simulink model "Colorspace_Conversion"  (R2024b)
settings: Solver=VariableStepAuto  StartTime=0.0  StopTime=10  RelTol=1e-3  EnableMultiTasking=on
undefined symbols (not defined in the file or in its folder): gray
libraries: ModelComposer x21, dspvision x1

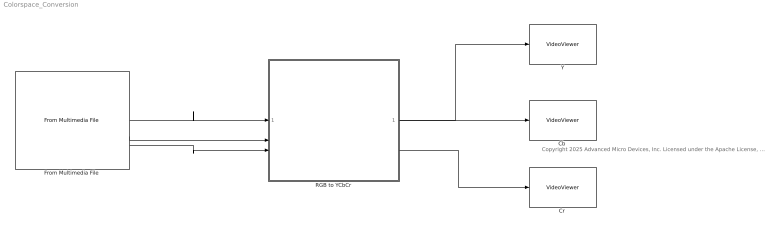
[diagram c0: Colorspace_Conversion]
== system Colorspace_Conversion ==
  note: Copyright 2025 Advanced Micro Devices, Inc. Licensed under the Apache License, Version 2.0 (the "License"); you may not use this file except in compliance with the License. You may obtain a copy of the License at http://www.apache.org/licenses/LICENSE-2.0 Unless required by applicable law or agreed to in writing, software distributed under the License is distributed on an "AS IS" BASIS, WITHOUT WARRANTIES OR CONDITIONS OF ANY KIND, either express or implied. See the License for the specific language governing permissions and limitations under the License.
  "Cb " : VideoViewer  colormapValue=gray(256)  FigPos=[23.4 519.6 487.2 356]
  "Cr " : VideoViewer  colormapValue=gray(256)  FigPos=[534.6 513.2 460.8 352]
  From Multimedia File : dspvision/From Multimedia File  inputFilename=visionface.avi  readRange=[1 Inf]  loop=on  numPlays=inf  outputStreams=Video only  videoDataType=single  audioDataType=int16  inheritSampleTime=on  userDefinedSampleTime=1/30  noAudioOutput=off  isIntensityVideo=off  fourcc=RGB  colorVideoFormat=Separate color signals  outputEOF=off  dataOrg=Column-major  audioFrameSize=1024  computeAudioFrameSize=off  outSamplingMode=Sample based
  RGB to YCbCr : Subsystem
  Y : VideoViewer  colormapValue=gray(256)  FigPos=[1016.2 530.8 471.2 368.8]
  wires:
  From Multimedia File/2 -> RGB to YCbCr/2(G)
  From Multimedia File/3 -> RGB to YCbCr/3(B)
  From Multimedia File/1 -> RGB to YCbCr/1(R)
  RGB to YCbCr/1(Y) -> Y/1
  RGB to YCbCr/2(Cb) -> "Cb "/1
  RGB to YCbCr/3(Cr) -> "Cr "/1

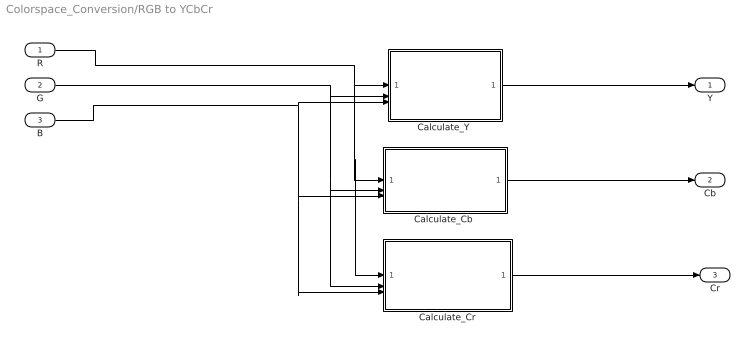
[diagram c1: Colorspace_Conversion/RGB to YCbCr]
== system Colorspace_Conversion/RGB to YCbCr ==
  R : Inport
  G : Inport  Port=2
  B : Inport  Port=3
  "Calculate_Cb " : Subsystem
  Calculate_Cr : Subsystem
  "Calculate_Y " : Subsystem
  Y : Outport
  Cb : Outport  Port=2
  Cr : Outport  Port=3
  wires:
  "Calculate_Y "/1(Out1) -> Y/1
  "Calculate_Cb "/1("Cb ") -> Cb/1
  Calculate_Cr/1(Cr) -> Cr/1
  R/1 -> Calculate_Cr/1("R "), "Calculate_Cb "/1("R "), "Calculate_Y "/1("R ")
  G/1 -> Calculate_Cr/2("G "), "Calculate_Cb "/2("G "), "Calculate_Y "/2("G ")
  B/1 -> Calculate_Cr/3(B), "Calculate_Cb "/3(B), "Calculate_Y "/3("B ")

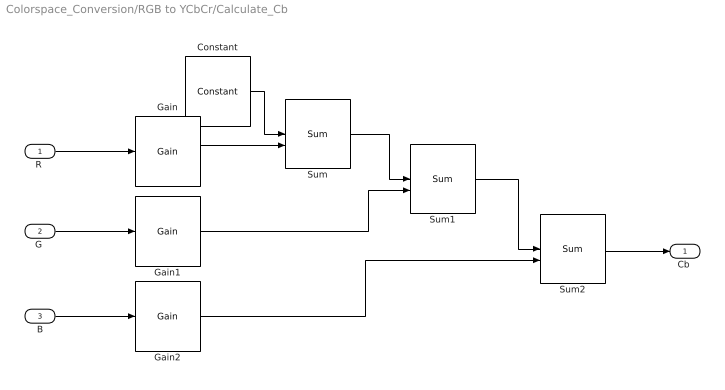
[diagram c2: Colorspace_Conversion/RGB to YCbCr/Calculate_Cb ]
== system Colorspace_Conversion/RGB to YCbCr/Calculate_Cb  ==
  "R " : Inport
  "G " : Inport  Port=2
  B : Inport  Port=3
  Constant : ModelComposer/Constant  Description=Performs multiplication  Value=128/255  SampleTime=-1  OutDataType=single  TypeExp=''  Signedness=Signed  WordLength=16  FractionalLength=0  RoundingMode=Truncation to minus infinity  OverflowMode=Wrap around
  Gain : ModelComposer/Gain  Description=Performs multiplication  Gain=-37.945/256  OutDataType=single  TypeExp=''  Signedness=Signed  WordLength=5  FractionalLength=4  RoundingMode=Truncation to minus infinity  OverflowMode=Wrap around  OutputTypeAsInput=on
  Gain1 : ModelComposer/Gain  Description=Performs multiplication  Gain=-74.494/256  OutDataType=single  TypeExp=''  Signedness=Signed  WordLength=5  FractionalLength=4  RoundingMode=Truncation to minus infinity  OverflowMode=Wrap around  OutputTypeAsInput=on
  Gain2 : ModelComposer/Gain  Description=Performs multiplication  Gain=112.439/256  OutDataType=single  TypeExp=''  Signedness=Signed  WordLength=5  FractionalLength=4  RoundingMode=Truncation to minus infinity  OverflowMode=Wrap around  OutputTypeAsInput=on
  Sum : ModelComposer/Sum
  Sum1 : ModelComposer/Sum
  Sum2 : ModelComposer/Sum
  "Cb " : Outport
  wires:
  Sum2/1 -> "Cb "/1
  "R "/1 -> Gain/1
  "G "/1 -> Gain1/1
  B/1 -> Gain2/1
  Constant/1 -> Sum/1
  Gain/1 -> Sum/2
  Sum/1 -> Sum1/1
  Gain1/1 -> Sum1/2
  Sum1/1 -> Sum2/1
  Gain2/1 -> Sum2/2

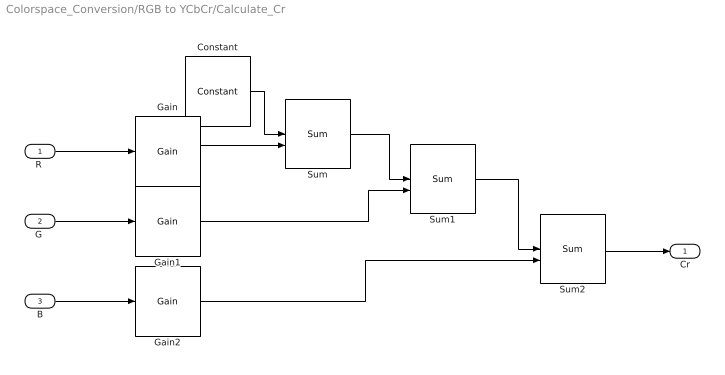
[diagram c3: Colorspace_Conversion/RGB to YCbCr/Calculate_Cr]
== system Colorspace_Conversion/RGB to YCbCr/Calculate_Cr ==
  "R " : Inport
  "G " : Inport  Port=2
  B : Inport  Port=3
  Constant : ModelComposer/Constant  Description=Performs multiplication  Value=128/255  SampleTime=-1  OutDataType=single  TypeExp=''  Signedness=Signed  WordLength=16  FractionalLength=0  RoundingMode=Truncation to minus infinity  OverflowMode=Wrap around
  Gain : ModelComposer/Gain  Description=Performs multiplication  Gain=112.439/256  OutDataType=single  TypeExp=''  Signedness=Signed  WordLength=5  FractionalLength=4  RoundingMode=Truncation to minus infinity  OverflowMode=Wrap around  OutputTypeAsInput=on
  Gain1 : ModelComposer/Gain  Description=Performs multiplication  Gain=-94.154/256  OutDataType=single  TypeExp=''  Signedness=Signed  WordLength=5  FractionalLength=4  RoundingMode=Truncation to minus infinity  OverflowMode=Wrap around  OutputTypeAsInput=on
  Gain2 : ModelComposer/Gain  Description=Performs multiplication  Gain=-18.285/256  OutDataType=single  TypeExp=''  Signedness=Signed  WordLength=5  FractionalLength=4  RoundingMode=Truncation to minus infinity  OverflowMode=Wrap around  OutputTypeAsInput=on
  Sum : ModelComposer/Sum
  Sum1 : ModelComposer/Sum
  Sum2 : ModelComposer/Sum
  Cr : Outport
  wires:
  Gain2/1 -> Sum2/2
  Sum1/1 -> Sum2/1
  Gain1/1 -> Sum1/2
  Sum/1 -> Sum1/1
  Gain/1 -> Sum/2
  Constant/1 -> Sum/1
  B/1 -> Gain2/1
  "G "/1 -> Gain1/1
  "R "/1 -> Gain/1
  Sum2/1 -> Cr/1

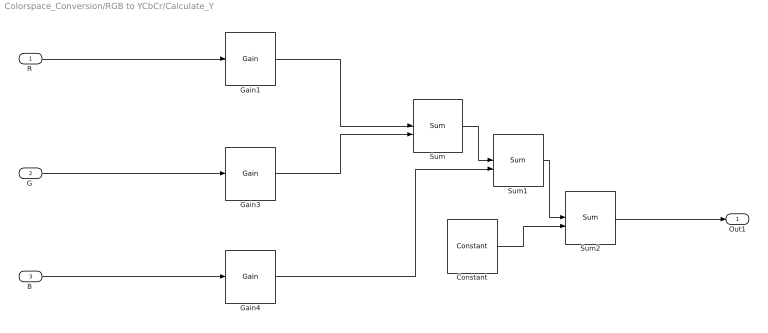
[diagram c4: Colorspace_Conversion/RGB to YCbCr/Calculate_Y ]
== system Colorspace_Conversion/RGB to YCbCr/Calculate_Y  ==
  "R " : Inport
  "G " : Inport  Port=2
  "B " : Inport  Port=3
  Constant : ModelComposer/Constant  Description=Performs multiplication  Value=16/255  SampleTime=-1  OutDataType=single  TypeExp=''  Signedness=Signed  WordLength=16  FractionalLength=0  RoundingMode=Truncation to minus infinity  OverflowMode=Wrap around
  Gain1 : ModelComposer/Gain  Description=Performs multiplication  Gain=65.738/256  OutDataType=single  TypeExp=''  Signedness=Signed  WordLength=5  FractionalLength=4  RoundingMode=Truncation to minus infinity  OverflowMode=Wrap around  OutputTypeAsInput=on
  Gain3 : ModelComposer/Gain  Description=Performs multiplication  Gain=129.057/256  OutDataType=single  TypeExp=''  Signedness=Signed  WordLength=5  FractionalLength=4  RoundingMode=Truncation to minus infinity  OverflowMode=Wrap around  OutputTypeAsInput=on
  Gain4 : ModelComposer/Gain  Description=Performs multiplication  Gain=25.064/256  OutDataType=single  TypeExp=''  Signedness=Signed  WordLength=5  FractionalLength=4  RoundingMode=Truncation to minus infinity  OverflowMode=Wrap around  OutputTypeAsInput=on
  Sum : ModelComposer/Sum
  Sum1 : ModelComposer/Sum
  Sum2 : ModelComposer/Sum
  Out1 : Outport
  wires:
  Sum/1 -> Sum1/1
  "R "/1 -> Gain1/1
  "B "/1 -> Gain4/1
  "G "/1 -> Gain3/1
  Gain1/1 -> Sum/1
  Gain3/1 -> Sum/2
  Gain4/1 -> Sum1/2
  Sum1/1 -> Sum2/1
  Constant/1 -> Sum2/2
  Sum2/1 -> Out1/1
